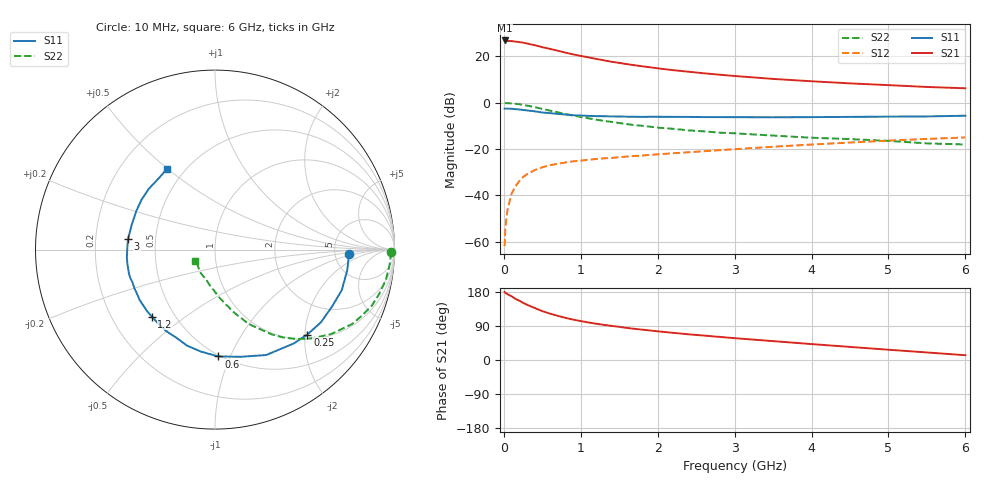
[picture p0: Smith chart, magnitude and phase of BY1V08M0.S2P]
! SIEMENS Small Signal Semiconductors
! BFY420
! Si NPN RF SIEGET Grounded Emitter Transistor in MICRO-X
! VCE = 1 V  IC = 8 mA
! Common Emitter S-Parameters:  October  1996
# GHz  S  MA  R  50
!  f  S11  S21  S12  S22
! GHz  MAG  ANG  MAG  ANG  MAG  ANG  MAG  ANG
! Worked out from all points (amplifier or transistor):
!   36 points, 10 MHz to 6 GHz, reference 50 ohm
!   highest |S21| = 26.9 dB at 10 MHz (marker M1)
!   |S21| within 3 dB of that: start of sweep to 514.1 MHz
!   unconditionally stable (mu >= 1): 2.586 GHz to end of sweep
!   at 250 MHz: K = 0.16, MSG = 29.0 dB, |S12| = -32.1 dB
!   at 1.4 GHz: K = 0.70, MSG = 20.8 dB, |S12| = -23.8 dB
!   at 6 GHz: K = 1.13, MAG = 8.4 dB, |S12| = -15.0 dB
!   S11 on the Smith chart (normalised r, x): 10 MHz: 6.79, -0.76; 250 MHz: 1.11, -2.06; 600 MHz: 0.49, -0.90; 1.2 GHz: 0.37, -0.38; 3 GHz: 0.35, +0.06; 6 GHz: 0.40, +0.50
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0.01  0.7462 -1.9  22.09 179.6  0.0008 96.3  0.9784 -0.9
0.02  0.7457 -4.0  22.07 177.0  0.0021 82.1  0.9798 -1.9
0.05  0.7457 -9.0  21.52 173.4  0.0051 88.6  0.9768 -5.0
0.1  0.7415 -17.8  21.43 168.2  0.0108 81.8  0.9667 -10.1
0.15  0.7252 -25.9  20.84 161.4  0.0156 76.9  0.9472 -15.2
0.2  0.7157 -34.5  20.39 156.6  0.0202 73.6  0.9277 -19.7
0.25  0.6991 -42.6  19.81 150.9  0.0249 69.3  0.8962 -24.4
0.3  0.6826 -50.0  19.01 145.9  0.0285 66.4  0.8692 -28.5
0.4  0.653 -64.1  17.48 137.4  0.035 60.8  0.801 -35.9
0.5  0.6144 -76.4  15.82 128.9  0.0404 56.0  0.7351 -42.2
0.6  0.5956 -88.2  14.52 122.4  0.0449 52.5  0.675 -47.6
0.8  0.5572 -106.3  12.08 111.3  0.0512 47.2  0.5712 -56.0
0.9  0.536 -113.7  11.06 106.6  0.0543 45.4  0.5289 -58.9
1.1  0.5196 -127.4  9.53 99.1  0.0589 43.6  0.4605 -65.0
1.2  0.5133 -133.3  8.838 95.7  0.0608 43.1  0.4315 -67.3
1.6  0.4991 -150.9  6.797 84.6  0.0688 40.9  0.3457 -75.1
2.2  0.495 -169.6  5.044 71.7  0.0811 39.8  0.2736 -84.0
3  0.4877 172.8  3.774 57.6  0.0993 38.0  0.2185 -93.7
3.5  0.4842 163.1  3.266 49.8  0.112 36.1  0.1952 -99.9
4.5  0.4946 145.9  2.615 34.5  0.1383 29.9  0.1638 -112.8
5.5  0.5059 128.4  2.189 19.9  0.1654 22.2  0.1325 -135.6
6  0.5241 120.5  2.048 12.6  0.178 17.9  0.1255 -150.8
